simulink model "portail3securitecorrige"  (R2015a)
settings: Solver=FixedStepDiscrete  StartTime=0.0  StopTime=inf  RelTol=1e-3
libraries: realtime_pacer_lib x1

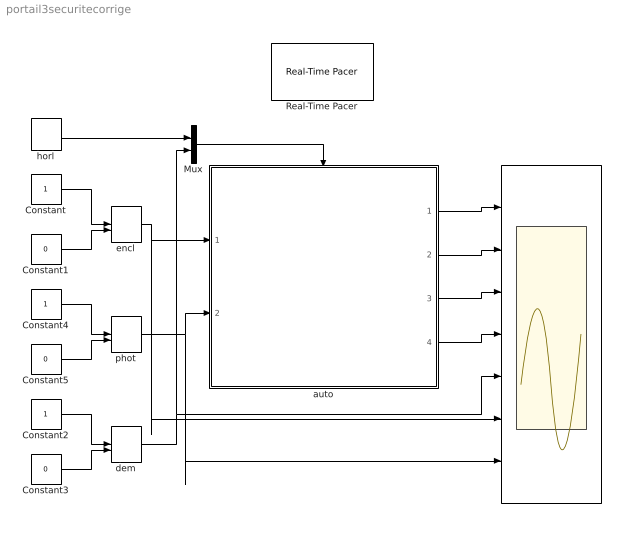
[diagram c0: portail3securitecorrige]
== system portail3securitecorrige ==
  " " : Scope  NumInputPorts=7
  Constant : Constant
  Constant1 : Constant  Value=0
  Constant2 : Constant
  Constant3 : Constant  Value=0
  Constant4 : Constant
  Constant5 : Constant  Value=0
  Mux : Mux  Inputs=2
  Real-Time Pacer : realtime_pacer_lib/Real-Time Pacer  simTimePerRealTime=1
  auto : Stateflow chart  TreatAsAtomicUnit=on
  dem : ManualSwitch  CurrentSetting=0
  encl : ManualSwitch  CurrentSetting=0
  horl : DiscretePulseGenerator  PulseType=Time based  Period=0.1  PulseWidth=5
  phot : ManualSwitch  CurrentSetting=0
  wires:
  Constant/1 -> encl/1
  Constant1/1 -> encl/2
  Constant2/1 -> dem/1
  Constant3/1 -> dem/2
  auto/1(CGV) -> " "/1
  auto/2(SGV) -> " "/2
  auto/4(SPV) -> " "/4
  encl/1 -> " "/6, auto/1(encl)
  dem/1 -> Mux/2, " "/5
  auto/3(CPV) -> " "/3
  horl/1 -> Mux/1
  Mux/1 -> auto/Trigger
  Constant4/1 -> phot/1
  Constant5/1 -> phot/2
  phot/1 -> " "/7, auto/2(phot)

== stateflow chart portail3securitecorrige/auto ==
  state portail_arrete
    du:CGV=0;
    SGV=0;
    CPV=0;
    SPV=0;
  state portail_marche_auto
    state ouverture
      du:CGV=150;
      SGV=0;
      CPV=150;
      SPV=0;
    state arret
      du:CGV=0;
      SGV=0;
      CPV=0;
      SPV=0;
    state fermeture
      state fermeture_G_V [parallel]
        state fermGV
          du:CGV=150;
          SGV=1;
        (default) -> fermGV
      state fermeture_P_V [parallel]
        state fermPV
          du:CPV=150;
          SPV=1;
        state attentePV
        (default) -> attentePV
        attentePV -> fermPV : after(2,sec)
    state securite
      du:CGV=0;
      SGV=0;
      CPV=0;
      SPV=0;
    state arretbis
      du:CGV=0;
      SGV=0;
      CPV=0;
      SPV=0;
    (default) -> arret
    arret -> ouverture : dem
    fermeture -> arret : after(5,sec)
    securite -> ouverture : [!phot]
    ouverture -> securite : [phot]
    ouverture -> arretbis : after(5,sec)
    fermeture -> securite : [phot]
    arretbis -> fermeture : after(4,sec)
  (default) -> portail_arrete
  portail_marche_auto -> portail_arrete : [!encl]
  portail_arrete -> portail_marche_auto : [encl]
  data: CGV output; SGV output; CPV output; SPV output; encl input; phot input
  events: input RISING_EDGE_EVENT; input RISING_EDGE_EVENT
